ORGANIZATION_BLOCK OB 86
TITLE = "Loss Of Rack Fault"
AUTHOR : Esposito
FAMILY : EGAL_srl
VERSION : 0.1


VAR_TEMP
  OB86_EV_CLASS : BYTE ;	//16#38/39 Event class 3
  OB86_FLT_ID : BYTE ;	//16#C1/C4/C5, Fault identification code
  OB86_PRIORITY : BYTE ;	//26/28 (Priority of 1 is lowest)
  OB86_OB_NUMBR : BYTE ;	//86 (Organization block 86, OB86)
  OB86_RESERVED_1 : BYTE ;	//Reserved for system
  OB86_RESERVED_2 : BYTE ;	//Reserved for system
  OB86_MDL_ADDR : WORD ;	//Depending on fault identification code
  OB86_RACKS_FLTD : ARRAY  [0 .. 31 ] OF BOOL ;	//Racks in fault
  OB86_DATE_TIME : DATE_AND_TIME ;	//Date and time OB86 started
END_VAR
BEGIN
NETWORK
TITLE =



END_ORGANIZATION_BLOCK

